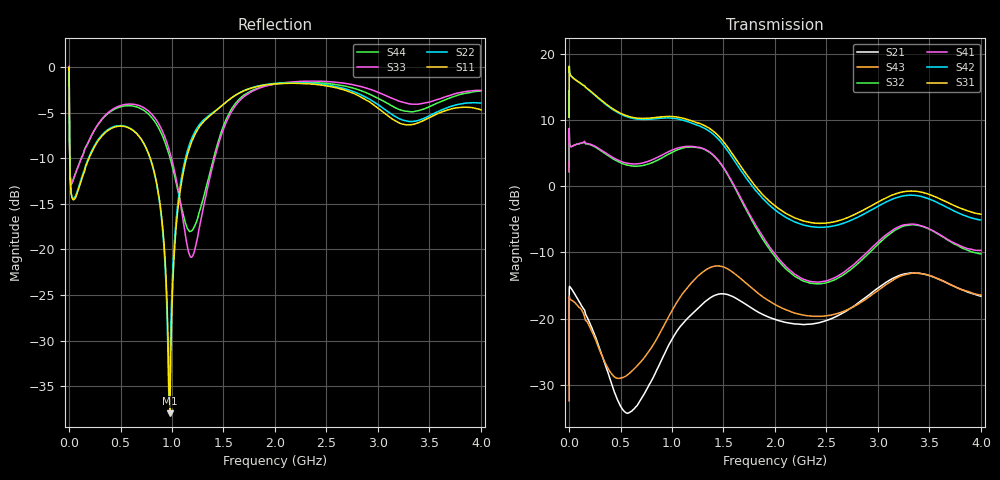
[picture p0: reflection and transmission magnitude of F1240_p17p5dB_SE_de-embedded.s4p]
! Integrated Device Technology
! Corporate Headquarters
! 6024 Silver Creek Valley Road
! San Jose, CA 95138  USA
! Phone:  1-408-284-8200
! Toll Free:  1-800-223-1366
! Webpage:  http://www.idt.com/
! Timing and RF Division
! 515 Groton Road, Suite 102
! Westford, MA 01886-6024
! Device:  F1240
! Description: Dual Intermediate Frequency Digital Variable Gain Amplifier
! Frequency:  10.0 -  500.00 MHz
! Package:  5x5 mm QFN Plastic Package: 32 pin
! Ports:  8 RF, 20 DC
!  Pin  1  = GA3 / Data  Pin 17  = RF OUT_B+
!  Pin  2  = GA4 / CLK  Pin 18  = RF OUT_B-
!  Pin  3  = GA5  Pin 19  = STBY_B
!  Pin  4  = VMODE  Pin 20  = Ground
!  Pin  5  = No Connect  Pin 21  = Ground
!  Pin  6  = GB5  Pin 22  = STB_A
!  Pin  7  = GB4  Pin 23  = RF OUT_A-  = Port 4
!  Pin  8  = GB3  Pin 24  = RF OUT_A+  = Port 3
!  Pin  9  = GB2  Pin 25  = GA0
!  Pin 10  = GB1  Pin 26  = ISET_A
!  Pin 11  = RF IN_B+  Pin 27  = VCC
!  Pin 12  = RF IN_B-  Pin 28  = Ground
!  Pin 13  = Ground  Pin 29  = RF IN_A-  = Port 2
!  Pin 14  = VCC  Pin 30  = RF IN_A+  = Port 1
!  Pin 15  = ISET_B  Pin 31  = GA1
!  Pin 16  = GB0  Pin 32  = GA2 / CSb
! Gain  = +19.5 dB
! State  = 1
! Voltage  = +5.00 V
! Current  = 85.292 mA (one channel only)
! Temperture  =  +25 C
! Test Date  =  2017-10-18
! Board  =  EB4031
! Data:  The device was measured on a custom evaluation board which has
!  individual transmission lines to the RF pins.  Data was collected
!  using a calibrated network analyzer.  The evaluation board was
!  de-embedded using Automatic Fixture Removal.
!  The reference plane is the edge of the package pin.
!  Only Channel A was measured.
!  This data is in single-ended operation.  If your needs are balanced
!  or differential S-parameters then this file needs to be used a
!  linear simulator.
! File Date:  2017-11-10  MJV
! Note:
!  Integrated Device Technology supplies this data as a sample of measured
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# Hz S dB R 100
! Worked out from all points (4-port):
!   410 points, 500 kHz to 4 GHz, reference 100 ohm
!   strongest paths, dB at 500 kHz, 930 MHz, 1.96 GHz, 2.98 GHz, 4 GHz:
!     S31: 10.4, 10.5, -2.5, -2.6, -4.2
!     S42: 10.4, 10.3, -3.1, -3.2, -5.1
!     S41: 2.2, 4.9, -9.5, -8.7, -9.7
!     S32: 2.2, 4.5, -9.8, -9.1, -10.2
!     S43: -32.4, -20.8, -17.5, -16.0, -16.5
!     S21: -30.1, -25.2, -19.9, -15.6, -16.6
!   lowest |S11| = -38.0 dB at 980 MHz (marker M1), VSWR 1.03, Z = 102 - j0.577 ohm
!   |S11| at or under -10 dB: 7.042 MHz to 193.6 MHz (186.5 MHz wide, 186 % of centre); 789.4 MHz to 1.14 GHz (350.2 MHz wide, 36.3 % of centre)
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500000  -0.29 -6.5  -29.94 18.7  -27.47 73.1  -62.67 64.4
        -30.07 18.6  -0.29 -6.5  -61.90 63.0  -27.47 74.3
        10.40 -105.5  2.17 72.6  -0.40 0.8  -32.43 -169.4
        2.18 73.6  10.38 -104.4  -32.44 -169.5  -0.41 3.1
3000000  -5.12 -51.7  -15.24 18.1  -20.46 10.8  -38.76 52.5
         -15.24 18.2  -5.09 -51.8  -38.76 52.4  -20.46 10.9
         17.76 -170.2  7.11 -2.0  -4.76 -47.0  -16.70 32.3
         7.11 -1.9  17.75 -170.1  -16.66 32.2  -4.82 -46.7
2.1e8  -9.58 -113.1  -20.94 -108.4  -23.35 -52.7  -33.61 7.1
       -20.98 -107.2  -9.42 -114.8  -33.62 7.2  -23.38 -52.6
       14.32 106.5  6.22 -60.0  -7.67 -80.7  -21.05 -115.9
       6.30 -60.0  14.26 105.7  -21.55 -114.2  -7.68 -80.0
5.6e8  -6.57 -173.5  -33.20 89.0  -24.96 -108.7  -27.60 -61.6
       -34.28 85.5  -6.53 -174.8  -27.77 -60.4  -25.12 -109.0
       10.61 20.0  3.19 -143.6  -4.05 -152.2  -27.86 85.9
       3.47 -144.5  10.48 18.8  -28.60 61.5  -4.22 -151.7
9.8e8  -37.99 -12.9  -21.71 -36.8  -22.02 165.2  -22.85 -161.0
       -23.66 -39.2  -32.99 -28.8  -23.20 -156.5  -22.47 164.7
       10.52 -82.0  4.93 125.2  -9.36 145.9  -18.58 -17.0
       5.29 120.3  10.27 -83.8  -19.35 -40.5  -9.93 151.6
1.51e9  -3.95 -141.7  -16.27 163.5  -28.49 40.3  -24.63 68.9
        -16.29 168.7  -3.96 -142.6  -24.62 74.7  -30.02 36.8
        6.50 118.7  2.48 -54.7  -6.48 -119.3  -12.05 160.2
        2.58 -59.7  5.96 117.3  -12.27 152.7  -6.13 -123.0
4e9  -4.66 -158.1  -16.66 56.3  -21.88 -37.2  -19.41 -48.3
     -16.62 55.6  -3.93 -151.6  -21.93 -29.5  -25.55 -19.9
     -4.24 -1.0  -10.24 -138.1  -2.54 -136.0  -14.82 89.6
     -9.72 -148.2  -5.12 8.0  -16.47 63.2  -2.59 -140.9
